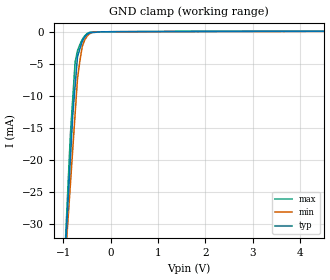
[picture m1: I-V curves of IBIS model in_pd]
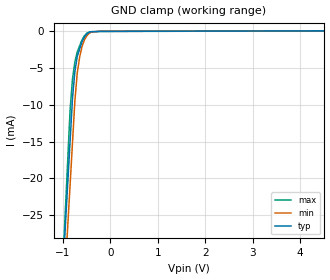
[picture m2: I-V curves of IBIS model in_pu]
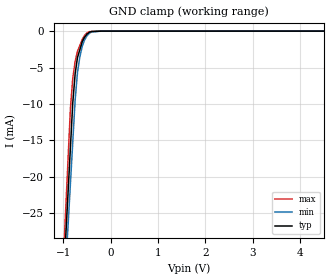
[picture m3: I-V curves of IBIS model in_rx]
[IBIS Ver]   3.2
[Comment Char] |_char
[File Name]   dir9001pw.ibs
[File Rev]   3.0
[Source]
| This model file was created by Teraspeed Consulting Group LLC
| (http://www.teraspeed.com/).
[Date]   06-18-2008
[Notes]   Quality Check of this IBIS model: Model Passes IBIS Check
   Model parses into ICX IS. Simulation done with Hyperlynx.
   1. MIN TYP MAX information is based on Temprature and Voltage
   characteristics only.
[Disclaimer]
| This model is designed as an aid for customers of Texas Instruments.
| TI and its licensors and suppliers make no warranties, either expressed
| or implied, with respect to this  model, including the warranties of
| merchantability or fitness for a particular purpose.
| The model is provided solely on an "as is" basis. The entire risk as to
| its quality and performance is with the customer.
[Copyright]
| (C) Copyright 2008 Texas Instruments Incorporated. All rights reserved.
[Component] DIR9001PW
[Manufacturer] TI
[Package]
| variable   typ   min   max
R_pkg  1.82E-01   1.70E-01  1.94E-01
L_pkg  4.90E-09   3.51E-09  6.35E-09
C_pkg  6.52E-13   5.62E-13  7.42E-13
[Pin] signal_name  model_name  R_pin  L_pin C_pin
1   _AUDIO  output  1.94E-01  6.35E-09  7.42E-13
2   FSOUT0  output  1.90E-01  5.86E-09  7.12E-13
3   FSOUT1  output  1.86E-01  5.37E-09  6.82E-13
4   SCKO   output  1.82E-01  4.89E-09  6.52E-13
5   VDD   POWER   1.78E-01  4.42E-09  6.22E-13
6   DGND   GND   1.74E-01  3.96E-09  5.92E-13
7   XTO   out_xto 1.70E-01  3.51E-09  5.62E-13
8   XTI   in_xti  1.70E-01  3.51E-09  5.62E-13
9   CLKST   output  1.74E-01  3.96E-09  5.92E-13
10   LRCKO   output  1.78E-01  4.42E-09  6.22E-13
11   BCKO   output  1.82E-01  4.89E-09  6.52E-13
12   DOUT   output  1.86E-01  5.37E-09  6.82E-13
13   PSCK0   in_pd   1.90E-01  5.86E-09  7.12E-13
14   PSCK1   in_pd   1.94E-01  6.21E-09  7.42E-13
15   COUT   output  1.94E-01  6.35E-09  7.42E-13
16   UOUT   output  1.90E-01  5.86E-09  7.12E-13
17   EMPH   output  1.86E-01  5.37E-09  6.82E-13
18   BFRAME  output  1.82E-01  4.89E-09  6.52E-13
19   RSV   in_pd   1.78E-01  4.42E-09  6.22E-13
20   RXIN   in_rx   1.74E-01  3.96E-09  5.92E-13
21   _RST   in_pu   1.70E-01  3.51E-09  5.62E-13
22   FILT   term   1.70E-01  3.51E-09  5.62E-13
23   AGND   GND   1.74E-01  3.96E-09  5.92E-13
24   VCC   POWER   1.78E-01  4.42E-09  6.22E-13
25   FMT0   in_pd   1.82E-01  4.89E-09  6.52E-13
26   FMT1   in_pd   1.86E-01  5.37E-09  6.82E-13
27   ERROR   output  1.90E-01  5.86E-09  7.12E-13
28   CKSEL   in_pd   1.94E-01  6.21E-09  7.42E-13
[Model] term
Model_type Terminator
C_comp 0.00000pF 0.00000pF 0.00000pF
| variable typ   min   max
[Voltage Range] 3.30000V 3.00000V 3.60000V
[POWER Clamp Reference] 3.30000V 3.00000V 3.60000V
[GND Clamp Reference] 0.00000V 0.00000V 0.00000V
[Temperature Range]   25   85   -40
| Models and submodels in the file (7): in_pd (Input), in_pu (Input), in_rx (Input), in_xti (Input), output (Output), out_xto (Output), term (Terminator)
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[Model] in_pd
Model_type Input
Vinl = 800.000mV
Vinh = 2.00000V
C_comp 717.0fF   717.0fF   717.0fF
| variable typ   min   max
[Voltage Range] 3.30000V 2.70000V 3.60000V
[POWER Clamp Reference] 3.30000V 2.70000V 3.60000V
[GND Clamp Reference] 0.00000V 0.00000V 0.00000V
[Temperature Range]   25   85   -40
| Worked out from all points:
|   GND clamp passes 1 mA (typ) near -0.56 V on its own axis
[GND Clamp]
-3.3V     -351.3mA   -292.6mA   -403.5mA
-850mV    -19.72mA   -23.75mA   -16mA
-800mV    -12.96mA   -18.26mA   -10.35mA
-750mV    -8.408mA   -12.78mA   -4.696mA
-700mV    -3.859mA   -7.29mA    -2.972mA
-650mV    -2.68mA    -4.55mA    -1.997mA
-600mV    -1.501mA   -2.323mA   -1.221mA
-550mV    -857.3uA   -1.314mA   -654.5uA
-450mV    -178.2uA   -340.5uA   -107.7uA
-350mV    -107.9uA   -52.19uA   -36.05uA
0V        0A         0A         0A
6.6V      104.9uA    80.32uA    96.04uA
[POWER Clamp]
-3.3V     0A         0A         0A
6.6V      0A         0A         0A
[Model] in_pu
Model_type Input
Vinl = 800.000mV
Vinh = 2.00000V
C_comp 1.020pF   1.020pF   1.020pF
| variable typ   min   max
[Voltage Range] 3.30000V 2.70000V 3.60000V
[POWER Clamp Reference] 3.30000V 2.70000V 3.60000V
[GND Clamp Reference] 0.00000V 0.00000V 0.00000V
[Temperature Range]   25   85   -40
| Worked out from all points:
|   GND clamp passes 1 mA (typ) near -0.56 V on its own axis
[GND Clamp]
-3.3V     -296.5mA   -297.3mA   -343.5mA
-850mV    -14.89mA   -20.8mA    -10.66mA
-800mV    -9.147mA   -15.16mA   -6.525mA
-750mV    -5.529mA   -9.516mA   -4.217mA
-700mV    -3.483mA   -5.731mA   -2.85mA
-650mV    -2.478mA   -3.59mA    -2.039mA
-600mV    -1.473mA   -2.148mA   -1.229mA
-550mV    -861.9uA   -1.255mA   -679.6uA
-450mV    -207.8uA   -345.7uA   -156uA
-400mV    -102.6uA   -152.6uA   -140.2uA
-200mV    -64.87uA   -37.37uA   -84.38uA
6.6V      38.15uA    32.16uA    40.13uA
[POWER Clamp]
-3.3V     0A         0A         0A
6.6V      0A         0A         0A
[Model] in_rx
Model_type Input
Vinl = 800.000mV
Vinh = 2.00000V
C_comp 1.510pF   1.510pF   1.510pF
| variable typ   min   max
[Voltage Range] 3.30000V 2.70000V 3.60000V
[POWER Clamp Reference] 3.30000V 2.70000V 3.60000V
[GND Clamp Reference] 0.00000V 0.00000V 0.00000V
[Temperature Range]   25   85   -40
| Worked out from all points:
|   GND clamp passes 1 mA (typ) near -0.56 V on its own axis
[GND Clamp]
-3.3V     -319.4mA   -303.7mA   -351.8mA
-850mV    -16.03mA   -20.98mA   -10.67mA
-800mV    -9.838mA   -15.21mA   -6.469mA
-750mV    -5.864mA   -9.445mA   -4.141mA
-700mV    -3.61mA    -5.642mA   -2.764mA
-650mV    -2.536mA   -3.512mA   -1.951mA
-600mV    -1.463mA   -2.081mA   -1.139mA
-550mV    -832uA     -1.199mA   -589.6uA
-450mV    -157.8uA   -300.2uA   -70.56uA
-400mV    -44.7uA    -112.2uA   -55.26uA
-200mV    -2.913uA   -2.9uA     -1.702uA
6.6V      4.444uA    5.78uA     3.431uA
[POWER Clamp]
-3.3V     0A         0A         0A
6.6V      0A         0A         0A
